|//////////////////////////////////////////////////////////////////////////////
|//////////////////////////////////////////////////////////////////////////////
|   @@@@@@@   @@@@@@@   @@@@@@@   @@@@@@@   @@@@@@@   @@@@@@   @@
|   @@@@@@@@@   @@@@@@@@@   @@@@@@@@@   @@@@@@@@@   @@@@@@@@@ @@@@@@@@  @
|   @@@   @@@ @@@   @@@ @@@   @@@   @@@ @@@   @@@@   @@@  @
|   @@   @@ @@   @@ @@@@@@@@@@@ @@@@@@@@@@@ @@   @@   @@ @@
|   @@@   @@@ @@   @@   @@@ @@@   @@   @@   @@ @@
|   @@@@@@@@@  @@   @@  @@@@@@@@@   @@@@@@@@@  @@   @@   @@ @@
|   @@@@@@@   @@   @@   @@@@@@@   @@@@@@@   @@   @@   @@ @@
|   IBIS Model of MC74VHC1GT126
|   Single Non-Inverting Buffer, 3-State, TTL Level
|   Package Type:  TSOP-5/SOT-23-5, CASE 483 (DT)
|   SC-88A/SC-70-5, CASE 419A-02 (DF)
|   SC-74A, CASE 318BQ (DBV)
|   SOT-553 (XV5), CASE 463B-01
|   SOT-953, CASE 527AE (P5)
|   UDFN6, CASE 517AQ (1.45 x 1.00 mm)
|   UDFN6, CASE 517AA (1.20 x 1.00 mm)
|   UDFN6, CASE 517BX (1.00 x 1.00 mm)
|   The model is covering the following Vccs:
|   2.0V, 2.5V, 3.3V, 5.0V
|//////////////////////////////////////////////////////////////////////////////
|//////////////////////////////////////////////////////////////////////////////
[IBIS Ver]   3.2
|   7.2 compatible
|//////////////////////////////////////////////////////////////////////////////
[Comment Char] |_char
|//////////////////////////////////////////////////////////////////////////////
[File Name]   74vhc1gt126_va_r0.ibs
|//////////////////////////////////////////////////////////////////////////////
[File Rev]   0.0
|   0.0 - February 29, 2024 - File created
|//////////////////////////////////////////////////////////////////////////////
[Date]   Feb 29, 2024
|//////////////////////////////////////////////////////////////////////////////
[Source]   From lab measurements and simulations at onsemi
|//////////////////////////////////////////////////////////////////////////////
[Notes]
   - The currents greater than +/- 100 mA are extrapolated
|//////////////////////////////////////////////////////////////////////////////
[Disclaimer]
   - onsemi Corporation hereby grants
   the user of this IBIS model a license to use this model
   under the following terms. This license is nonexclusive
   and nontransferable. Before using this IBIS model.
   After reading the terms and conditions of this license,
   the user either must accept these terms,
   or the IBIS model should be returned to onsemi within 30 days.
   - The user is hereby granted a license to use the IBIS model.
   This shall not be construed as a right to sell,
   or otherwise profit either by leasing or renting this software.
   - The user may modify the IBIS model to suit his specific
   applications but rights to derivative works and such
   modifications shall belong to onsemi.
   - This IBIS model is provided on an "as is" basis.
   onsemi makes absolutely no warranty with respect
   to the information contained herein.
   By use of this IBIS model, the user assumes full risk as to the
   quality and suitablility of the model to his particular use,
   and by using this model assumes the entire risk.
   Under all circumstances the user shall not hold
   onsemi liable in any way for the results obtained.
   onsemi reserves the right to make to improve
   the model for reliability, function, or design.
   onsemi does not convey any license under patent
   rights or any other intellectual property rights,
   including those of third parties.
   - onsemi is not obligated to provide maintenance
   or support for the licensed IBIS model.
   - Cont onsemi at ATTN:LOGIC APPLICATIONS/IBIS MODEL.
   5701 N Pima Rd, Scottsdale, AZ 85250
|//////////////////////////////////////////////////////////////////////////////
[Copyright]   (c) 2024 onsemi Corp.
|//////////////////////////////////////////////////////////////////////////////
|//////////////////////////////////////////////////////////////////////////////
[Component]   M74VHC1GT126DT1G-Q
|//////////////////////////////////////////////////////////////////////////////
[Manufacturer]  onsemi
|   Data Sheet:   MC74VHC1G126/D, Rev. 26,  Jan, 2024
|//////////////////////////////////////////////////////////////////////////////
[Package]
| TSOP-5/SOT-23-5
|   DT SUFFIX
|   CASE 483
| variable   typ   min   max
R_pkg   0.02532   0.0216   0.0295
L_pkg   1.52928nH   1.3125nH   1.9067nH
C_pkg   0.15688pF   0.1108pF   0.2403pF
|//////////////////////////////////////////////////////////////////////////////
[Pin]   signal_name   model_name   R_pin   L_pin   C_pin
1   OE   In   0.0216   1.5112nH   0.1443pF
2   A   In   0.0237   1.3125nH   0.1382pF
3   GND   GND   0.0295   1.9067nH   0.2403pF
4   Y   Out   0.0266   1.5415nH   0.1508pF
5   VCC   POWER   0.0252   1.3745nH   0.1108pF
|//////////////////////////////////////////////////////////////////////////////
|//////////////////////////////////////////////////////////////////////////////
[Component]   M74VHC1GT126DF1G
|//////////////////////////////////////////////////////////////////////////////
[Manufacturer]  onsemi
|   Data Sheet:   MC74VHC1G126/D, Rev. 26,  Jan, 2024
|//////////////////////////////////////////////////////////////////////////////
[Package]
| SC-88A / SC-70-5
|   DF SUFFIX
|   CASE 419A-02
| variable   typ   min   max
R_pkg   0.0201   0.0170   0.0250
L_pkg   0.9982nH   0.8810nH   1.0690nH
C_pkg   0.1466pF   0.1187pF   0.2051pF
|//////////////////////////////////////////////////////////////////////////////
[Pin]   signal_name   model_name   R_pin   L_pin   C_pin
1   OE   In   0.0191   1.0690nH   0.1625pF
2   A   In   0.0187   0.8810nH   0.1217pF
3   GND   GND   0.0170   1.0315nH   0.2051pF
4   Y   Out   0.0207   0.9600nH   0.1249pF
5   VCC   POWER   0.0250   1.0497nH   0.1187pF
|//////////////////////////////////////////////////////////////////////////////
|//////////////////////////////////////////////////////////////////////////////
[Component]   M74VHC1GT126DF2G
|//////////////////////////////////////////////////////////////////////////////
[Manufacturer]  onsemi
|   Data Sheet:   MC74VHC1G126/D, Rev. 26,  Jan, 2024
|//////////////////////////////////////////////////////////////////////////////
[Package]
R_pkg   0.0201   0.0170   0.0250
L_pkg   0.9982nH   0.8810nH   1.0690nH
C_pkg   0.1466pF   0.1187pF   0.2051pF
|//////////////////////////////////////////////////////////////////////////////
[Pin]   signal_name   model_name   R_pin   L_pin   C_pin
1   OE   In   0.0191   1.0690nH   0.1625pF
2   A   In   0.0187   0.8810nH   0.1217pF
3   GND   GND   0.0170   1.0315nH   0.2051pF
4   Y   Out   0.0207   0.9600nH   0.1249pF
5   VCC   POWER   0.0250   1.0497nH   0.1187pF
|//////////////////////////////////////////////////////////////////////////////
|//////////////////////////////////////////////////////////////////////////////
[Component]   M74VHC1GT126DF1G-Q
|//////////////////////////////////////////////////////////////////////////////
[Manufacturer]  onsemi
|   Data Sheet:   MC74VHC1G126/D, Rev. 26,  Jan, 2024
|//////////////////////////////////////////////////////////////////////////////
[Package]
R_pkg   0.0201   0.0170   0.0250
L_pkg   0.9982nH   0.8810nH   1.0690nH
C_pkg   0.1466pF   0.1187pF   0.2051pF
|//////////////////////////////////////////////////////////////////////////////
[Pin]   signal_name   model_name   R_pin   L_pin   C_pin
1   OE   In   0.0191   1.0690nH   0.1625pF
2   A   In   0.0187   0.8810nH   0.1217pF
3   GND   GND   0.0170   1.0315nH   0.2051pF
4   Y   Out   0.0207   0.9600nH   0.1249pF
5   VCC   POWER   0.0250   1.0497nH   0.1187pF
|//////////////////////////////////////////////////////////////////////////////
|//////////////////////////////////////////////////////////////////////////////
[Component]   M74VHC1GT126DF2G-Q
|//////////////////////////////////////////////////////////////////////////////
[Manufacturer]  onsemi
|   Data Sheet:   MC74VHC1G126/D, Rev. 26,  Jan, 2024
|//////////////////////////////////////////////////////////////////////////////
[Package]
R_pkg   0.0201   0.0170   0.0250
L_pkg   0.9982nH   0.8810nH   1.0690nH
C_pkg   0.1466pF   0.1187pF   0.2051pF
|//////////////////////////////////////////////////////////////////////////////
[Pin]   signal_name   model_name   R_pin   L_pin   C_pin
1   OE   In   0.0191   1.0690nH   0.1625pF
2   A   In   0.0187   0.8810nH   0.1217pF
3   GND   GND   0.0170   1.0315nH   0.2051pF
4   Y   Out   0.0207   0.9600nH   0.1249pF
5   VCC   POWER   0.0250   1.0497nH   0.1187pF
|//////////////////////////////////////////////////////////////////////////////
|//////////////////////////////////////////////////////////////////////////////
[Component]   MC74VHC1GT126DBVT1G
|//////////////////////////////////////////////////////////////////////////////
[Manufacturer]  onsemi
|   Data Sheet:   MC74VHC1G126/D, Rev. 26,  Jan, 2024
|//////////////////////////////////////////////////////////////////////////////
[Package]
|  SC-74A
| DBV SUFFIX
| CASE 318BQ
| variable   typ   min   max
R_pkg   0.0710   0.0522   0.0935
L_pkg   1.2331nH   1.0634nH   1.4484nH
C_pkg   0.1280pF   0.1167pF   0.1367pF
|//////////////////////////////////////////////////////////////////////////////
[Pin]   signal_name   model_name   R_pin   L_pin   C_pin
1   OE   In   0.0522   1.0634nH   0.1235pF
2   A   In   0.0588   1.1995nH   0.1367pF
3   GND   GND   0.0828   1.3327nH   0.1351pF
4   Y   Out   0.0935   1.4484nH   0.1279pF
5   VCC   POWER   0.0679   1.1215nH   0.1167pF
|//////////////////////////////////////////////////////////////////////////////
|//////////////////////////////////////////////////////////////////////////////
[Component]   MC74VHC1GT126P5T5G
|//////////////////////////////////////////////////////////////////////////////
[Manufacturer]  onsemi
|   Data Sheet:   MC74VHC1G126/D, Rev. 26,  Jan, 2024
|//////////////////////////////////////////////////////////////////////////////
[Package]
|  SOT-953
| P5  SUFFIX
| CASE 527AE
| variable   typ   min   max
R_pkg   0.0786   0.0731   0.0817
L_pkg   1.1377nH   1.0330nH   1.1757nH
C_pkg   0.0487pF   0.0295pF   0.0642pF
|//////////////////////////////////////////////////////////////////////////////
[Pin]   signal_name   model_name   R_pin   L_pin   C_pin
1   A   In   0.0817   1.1757nH   0.0433pF
2   GND   GND   0.0731   1.0330nH   0.0295pF
3   OE   In   0.0805   1.1531nH   0.0500pF
4   Y   Out   0.0789   1.1637nH   0.0642pF
5   VCC   POWER   0.0787   1.1630nH   0.0567pF
|//////////////////////////////////////////////////////////////////////////////
|//////////////////////////////////////////////////////////////////////////////
[Component]   MC74VHC1GT126XV5T2G
|//////////////////////////////////////////////////////////////////////////////
[Manufacturer]  onsemi
|   Data Sheet:   MC74VHC1G126/D, Rev. 26,  Jan, 2024
|//////////////////////////////////////////////////////////////////////////////
[Package]
|  SOT-553
| XV5 SUFFIX
| CASE 463B-01
| variable   typ   min   max
R_pkg   0.0321   0.0287   0.0357
L_pkg   0.9169nH   0.7230nH   1.1357nH
C_pkg   0.2220pF   0.1035pF   0.3741pF
|//////////////////////////////////////////////////////////////////////////////
[Pin]   signal_name   model_name   R_pin   L_pin   C_pin
1   OE   In   0.0341   0.7230nH   0.1035pF
2   A   In   0.0287   0.8933nH   0.2377pF
3   GND   GND   0.0290   1.0725nH   0.3741pF
4   Y   Out   0.0357   0.7602nH   0.1139pF
5   VCC   POWER   0.0330   1.1357nH   0.2807pF
|//////////////////////////////////////////////////////////////////////////////
|//////////////////////////////////////////////////////////////////////////////
[Component]   MC74VHC1GT126MU1TCG
|//////////////////////////////////////////////////////////////////////////////
[Manufacturer]  onsemi
|   Data Sheet:   MC74VHC1G126/D, Rev. 26,  Jan, 2024
|//////////////////////////////////////////////////////////////////////////////
[Package]
|   UDFN-6
| 1.45 x 1.0
| CASE 517AQ
| variable   typ   min   max
R_pkg   0.0499   0.0010   0.0568
L_pkg   0.4063nH   0.0145nH   0.4786nH
C_pkg   0.1074pF   0.0765pF   0.1119pF
|//////////////////////////////////////////////////////////////////////////////
[Pin]   signal_name   model_name   R_pin   L_pin   C_pin
1   OE   In   0.0568   0.4786nH   0.1119pF
2   A   In   0.0469   0.3812nH   0.1077pF
3   GND   GND   0.0541   0.4521nH   0.1099pF
4   Y   Out   0.0513   0.4206nH   0.1072pF
5   NC   NC   0.0010   0.0145nH   0.0765pF
6   VCC   POWER   0.0484   0.3921nH   0.1051pF
|//////////////////////////////////////////////////////////////////////////////
|//////////////////////////////////////////////////////////////////////////////
[Component]   MC74VHC1GT126MU2TCG
|//////////////////////////////////////////////////////////////////////////////
[Manufacturer]  onsemi
|   Data Sheet:   MC74VHC1G126/D, Rev. 26,  Jan, 2024
|//////////////////////////////////////////////////////////////////////////////
[Package]
|  UDFN-6
| 1.2 x 1.0
| CASE 517AA
| variable   typ   min   max
R_pkg   0.0380   0.0007   0.0502
L_pkg   0.3514nH   0.0262nH   0.4657nH
C_pkg   0.1033pF   0.0765pF   0.1113pF
|//////////////////////////////////////////////////////////////////////////////
[Pin]   signal_name   model_name   R_pin   L_pin   C_pin
1   OE   In   0.0495   0.4460nH   0.1109pF
2   A   In   0.0407   0.3641nH   0.1069pF
3   GND   GND   0.0492   0.4551nH   0.1110pF
4   Y   Out   0.0502   0.4657nH   0.1113pF
5   NC   NC   0.0007   0.0262nH   0.0765pF
6   VCC   POWER   0.0461   0.4205nH   0.1085pF
|//////////////////////////////////////////////////////////////////////////////
|//////////////////////////////////////////////////////////////////////////////
[Component]   MC74VHC1GT126MU3TCG
|//////////////////////////////////////////////////////////////////////////////
[Manufacturer]  onsemi
|   Data Sheet:   MC74VHC1G126/D, Rev. 26,  Jan, 2024
|//////////////////////////////////////////////////////////////////////////////
[Package]
|  UDFN-6
| 1.0 x 1.0
| CASE 517BX
| variable   typ   min   max
R_pkg   0.0419   0.0344   0.0490
L_pkg   0.4237nH   0.3470nH   0.5107nH
C_pkg   0.1104pF   0.1061pF   0.1153pF
|//////////////////////////////////////////////////////////////////////////////
[Pin]   signal_name   model_name   R_pin   L_pin   C_pin
1   OE   In   0.0421   0.4133nH   0.1099pF
2   A   In   0.0344   0.3470nH   0.1061pF
3   GND   GND   0.0443   0.4580nH   0.1121pF
4   Y   Out   0.0490   0.5107nH   0.1153pF
5   NC   NC   0.0004   0.0379nH   0.0765pF
6   VCC   POWER   0.0438   0.4489nH   0.1118pF
|//////////////////////////////////////////////////////////////////////////////
|//////////////////////////////////////////////////////////////////////////////
[Model Selector]   In
In_20   Vcc = 2.00
In_25   Vcc = 2.50
In_33   Vcc = 3.30
In_50   Vcc = 5.00
|//////////////////////////////////////////////////////////////////////////////
[Model Selector]   Out
Out_20   Vcc = 2.00
Out_25   Vcc = 2.50
Out_33   Vcc = 3.30
Out_50   Vcc = 5.00
| Models and submodels in the file (8): In_20 (Input), Out_20 (3-state), In_25 (Input), Out_25 (3-state), In_33 (Input), Out_33 (3-state), In_50 (Input), Out_50 (3-state)
